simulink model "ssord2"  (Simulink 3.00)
settings: Solver=ode45  StartTime=0.0  StopTime=5.0  RelTol=1e-3

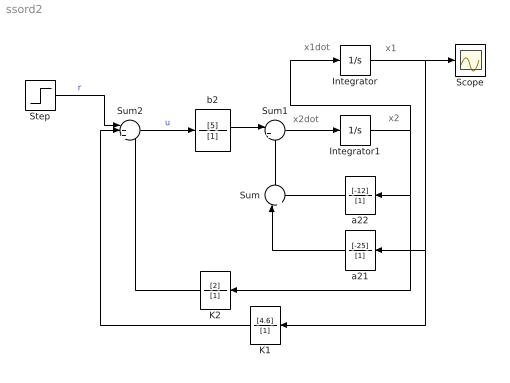
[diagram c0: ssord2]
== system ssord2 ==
  note: x1dot
  note: x2dot
  note: x1
  note: x2
  Integrator : Integrator  ExternalReset=none  InitialConditionSource=internal  InitialCondition=0  LimitOutput=off  UpperSaturationLimit=inf  LowerSaturationLimit=-inf  ShowSaturationPort=off  ShowStatePort=off  AbsoluteTolerance=auto
  Integrator1 : Integrator  ExternalReset=none  InitialConditionSource=internal  InitialCondition=0  LimitOutput=off  UpperSaturationLimit=inf  LowerSaturationLimit=-inf  ShowSaturationPort=off  ShowStatePort=off  AbsoluteTolerance=auto
  K1 : TransferFcn  Orientation=left  Numerator=[4.6]  Denominator=[1]
  K2 : TransferFcn  Orientation=left  Numerator=[2]  Denominator=[1]
  Scope : Scope
  Step : Step  Time=0  Before=0  After=1  SampleTime=0.001
  Sum : Sum  Orientation=up  Inputs=|++  SaturateOnIntegerOverflow=on
  Sum1 : Sum  Inputs=|++  SaturateOnIntegerOverflow=on
  Sum2 : Sum  Inputs=|+++  SaturateOnIntegerOverflow=on
  a21 : TransferFcn  Orientation=left  Numerator=[-25]  Denominator=[1]
  a22 : TransferFcn  Orientation=left  Numerator=[-12]  Denominator=[1]
  b2 : TransferFcn  Numerator=[5]  Denominator=[1]
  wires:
  a22/1 -> Sum/2
  a21/1 -> Sum/1
  Integrator1/1 -> Integrator/1, a22/1, K2/1
  Sum/1 -> Sum1/2
  Sum1/1 -> Integrator1/1
  b2/1 -> Sum1/1
  Integrator/1 -> Scope/1, a21/1, K1/1
  Sum2/1 -> b2/1  "u"
  K2/1 -> Sum2/3
  K1/1 -> Sum2/2
  Step/1 -> Sum2/1  "r"
